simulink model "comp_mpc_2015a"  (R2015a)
settings: Solver=ode45  StartTime=0.0  StopTime=120  FixedStep=0.025  MaxStep=0.5  MinStep=0.03  RelTol=1e-6
InitFcn:
  | X_init
  | X_init2
  | Xinit_inter
StopFcn:
  | finalplot
  | finalplot2
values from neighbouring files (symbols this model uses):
  Xinit = [97004.3048907971    [X_init.m]
  Xinit2 = [155100    [X_init2.m]
libraries: simulink x4

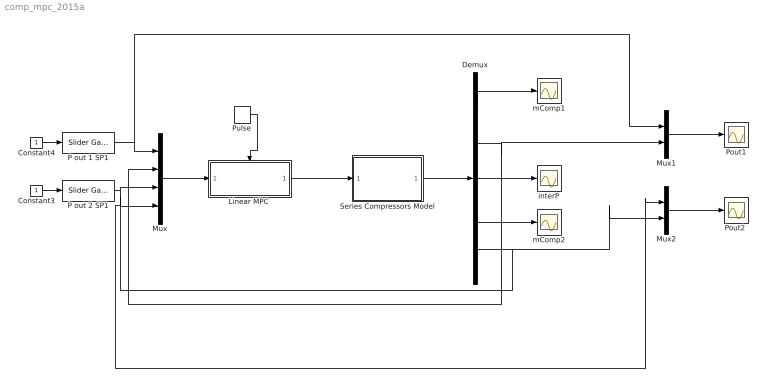
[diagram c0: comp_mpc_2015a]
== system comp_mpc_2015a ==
  Constant3 : Constant
  Constant4 : Constant
  Demux : Demux  Outputs=5
  "Linear MPC " : Subsystem  TreatAsAtomicUnit=on
  Mux : Mux
  Mux1 : Mux  Inputs=2
  Mux2 : Mux  Inputs=2
  P out 1 SP1 : simulink/Math Operations/Slider Gain  low=0  gain=173100  high=200000
  P out 2 SP1 : simulink/Math Operations/Slider Gain  low=0  gain=220000  high=2220000
  Pout1 : Scope
  "Pout2 " : Scope
  Pulse : DiscretePulseGenerator  PulseType=Time based  Period=0.5  PulseWidth=5
  Series Compressors Model : Subsystem
  interP : Scope
  mComp1 : Scope
  mComp2 : Scope
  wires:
  Demux/1 -> mComp1/1
  Demux/2 -> Mux1/2, Mux/2
  Demux/3 -> interP/1
  Demux/4 -> mComp2/1
  Demux/5 -> Mux2/2, Mux/4
  Pulse/1 -> "Linear MPC "/Trigger
  Mux/1 -> "Linear MPC "/1(In1)
  "Linear MPC "/1(Out1) -> Series Compressors Model/1(In1)
  Series Compressors Model/1(Out1) -> Demux/1
  Constant4/1 -> P out 1 SP1/1
  Constant3/1 -> P out 2 SP1/1
  P out 1 SP1/1 -> Mux1/1, Mux/1
  P out 2 SP1/1 -> Mux2/1, Mux/3
  Mux1/1 -> Pout1/1
  Mux2/1 -> "Pout2 "/1

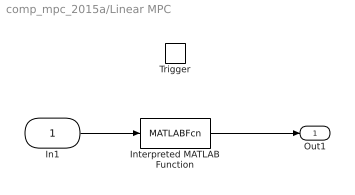
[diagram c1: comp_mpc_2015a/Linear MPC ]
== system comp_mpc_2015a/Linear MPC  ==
  In1 : Inport
  Trigger : TriggerPort
  Interpreted MATLAB Function : MATLABFcn  MATLABFcn=mpc_  Output1D=off
  Out1 : Outport
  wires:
  In1/1 -> Interpreted MATLAB Function/1
  Interpreted MATLAB Function/1 -> Out1/1

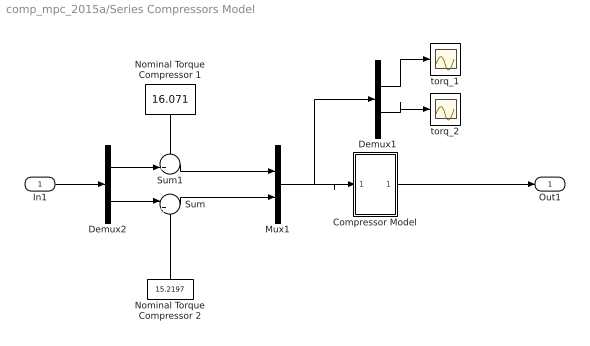
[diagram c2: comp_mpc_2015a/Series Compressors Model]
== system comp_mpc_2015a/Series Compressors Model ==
  In1 : Inport
  Compressor Model : Subsystem
  Demux1 : Demux  Outputs=2
  Demux2 : Demux  Outputs=2
  Mux1 : Mux  Inputs=2
  Nominal Torque Compressor 1 : Constant  Value=16.071
  Nominal Torque Compressor 2 : Constant  Value=15.2197
  Sum : Sum  Inputs=|++
  Sum1 : Sum  Inputs=++|
  torq_1 : Scope
  torq_2 : Scope
  Out1 : Outport
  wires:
  Demux1/2 -> torq_2/1
  Demux1/1 -> torq_1/1
  In1/1 -> Demux2/1
  Demux2/2 -> Sum/1
  Demux2/1 -> Sum1/2
  Sum/1 -> Mux1/2
  Sum1/1 -> Mux1/1
  Nominal Torque Compressor 1/1 -> Sum1/1
  Nominal Torque Compressor 2/1 -> Sum/2
  Mux1/1 -> Compressor Model/1(In1), Demux1/1
  Compressor Model/1(Out1) -> Out1/1

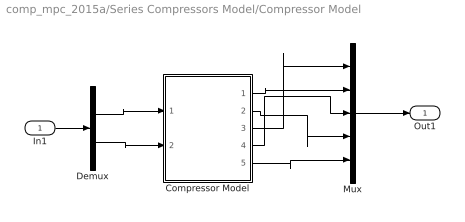
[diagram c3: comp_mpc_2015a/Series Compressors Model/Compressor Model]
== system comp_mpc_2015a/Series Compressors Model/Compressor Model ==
  In1 : Inport
  Compressor Model : Subsystem
  Demux : Demux  Outputs=2
  Mux : Mux  Inputs=5
  Out1 : Outport  PortDimensions=5
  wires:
  Compressor Model/4(iPres) -> Mux/3
  Mux/1 -> Out1/1
  Compressor Model/5(pout2) -> Mux/5
  Compressor Model/2(mcomp2) -> Mux/4
  Compressor Model/1(pout1) -> Mux/2
  Compressor Model/3(mcomp1) -> Mux/1
  Demux/1 -> Compressor Model/1(Torque 1)
  In1/1 -> Demux/1
  Demux/2 -> Compressor Model/2(torque 2)

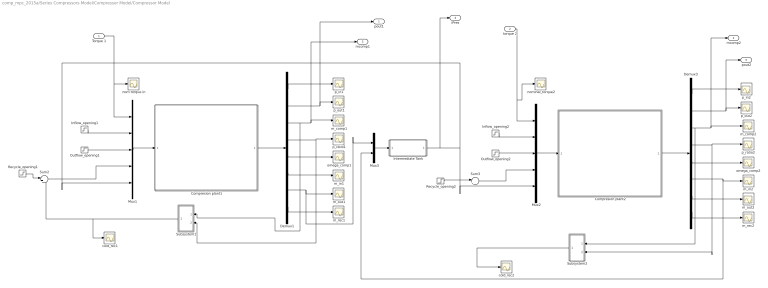
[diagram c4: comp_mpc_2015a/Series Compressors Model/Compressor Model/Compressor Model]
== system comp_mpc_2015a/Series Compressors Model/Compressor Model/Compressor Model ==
  Torque 1 : Inport
  torque 2 : Inport  Port=2
  Compresion plant1 : Subsystem
  Compresion plant2 : Subsystem
  Demux1 : Demux  Outputs=8
  Demux3 : Demux  Outputs=8
  Inflow_opening1 : Step  Time=0  Before=0.4541  After=0.4541  SampleTime=0
  Inflow_opening2 : Step  Time=25  Before=0.4541  After=0.4541  SampleTime=0
  Intermediate Tank : Subsystem
  Mux1 : Mux  Inputs=5
  Mux2 : Mux  Inputs=5
  Mux3 : Mux  Inputs=2
  Outflow_opening1 : Step  Time=10  Before=0.46  After=.29  SampleTime=0
  Outflow_opening2 : Step  Time=35  Before=0.46  After=.35  SampleTime=0
  Recycle_opening1 : Step  Time=2.05  After=0  SampleTime=0
  Recycle_opening2 : Step  Time=2.05  After=0  SampleTime=0
  Subsystem1 : Subsystem
  Subsystem2 : Subsystem
  Sum2 : Sum  Inputs=|++
  Sum3 : Sum  Inputs=|++
  cold_rec1 : Scope
  cold_rec2 : Scope
  m_comp1 : Scope
  m_comp2 : Scope
  m_in1 : Scope
  m_in2 : Scope
  m_out1 : Scope
  m_out2 : Scope
  m_rec1 : Scope
  m_rec2 : Scope
  nom torque in : Scope
  nominal_torque2 : Scope
  omega_comp1 : Scope
  omega_comp2 : Scope
  p_in1 : Scope
  p_in2 : Scope
  p_out1 : Scope
  p_out2 : Scope
  p_ratio1 : Scope
  p_ratio2 : Scope
  pout1 : Outport
  mcomp2 : Outport  Port=2
  mcomp1 : Outport  Port=3
  iPres : Outport  Port=4
  pout2 : Outport  Port=5
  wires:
  Sum3/1 -> Mux2/4
  Demux3/3 -> mcomp2/1, m_comp2/1, Subsystem2/1(In1)
  Demux3/4 -> Subsystem2/2(In2), p_ratio2/1
  Subsystem2/1(Out2) -> cold_rec2/1
  Torque 1/1 -> Mux1/1, nom torque in/1
  torque 2/1 -> Mux2/1, nominal_torque2/1
  Compresion plant1/1(Out1) -> Demux1/1
  Mux1/1 -> Compresion plant1/1(In1)
  Demux1/5 -> omega_comp1/1
  Demux1/6 -> m_in1/1
  Demux1/7 -> Mux3/1, m_out1/1
  Demux1/1 -> p_in1/1
  Demux1/2 -> pout1/1, p_out1/1
  Demux1/8 -> m_rec1/1
  Inflow_opening1/1 -> Mux1/2
  Compresion plant2/1(Out1) -> Demux3/1
  Mux2/1 -> Compresion plant2/1(In1)
  Demux3/5 -> omega_comp2/1
  Outflow_opening2/1 -> Mux2/3
  Demux3/6 -> Mux3/2, m_in2/1
  Demux3/7 -> m_out2/1
  Demux3/2 -> pout2/1, p_out2/1
  Demux3/8 -> m_rec2/1
  Outflow_opening1/1 -> Mux1/3
  Inflow_opening2/1 -> Mux2/2
  Mux3/1 -> Intermediate Tank/1(In1)
  Intermediate Tank/1(Out1) -> iPres/1, Mux2/5, Mux1/5
  Demux1/3 -> mcomp1/1, m_comp1/1, Subsystem1/1(In1)
  Demux1/4 -> p_ratio1/1, Subsystem1/2(In2)
  Subsystem1/1(Out2) -> Sum2/2, cold_rec1/1
  Recycle_opening1/1 -> Sum2/1
  Sum2/1 -> Mux1/4
  Recycle_opening2/1 -> Sum3/1
  Demux3/1 -> p_in2/1

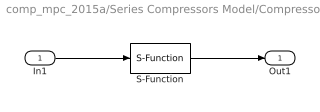
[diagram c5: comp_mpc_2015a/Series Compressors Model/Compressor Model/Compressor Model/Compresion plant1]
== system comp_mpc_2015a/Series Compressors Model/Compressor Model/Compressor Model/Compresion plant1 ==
  In1 : Inport
  S-Function : S-Function  FunctionName=comp_plant  Parameters=[],Xinit
  Out1 : Outport
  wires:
  S-Function/1 -> Out1/1
  In1/1 -> S-Function/1

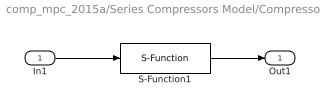
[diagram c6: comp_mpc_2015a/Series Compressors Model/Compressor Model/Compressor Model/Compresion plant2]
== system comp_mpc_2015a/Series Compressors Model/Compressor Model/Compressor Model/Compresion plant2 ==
  In1 : Inport
  S-Function1 : S-Function  FunctionName=comp_plant2  Parameters=[],Xinit2
  Out1 : Outport
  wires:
  S-Function1/1 -> Out1/1
  In1/1 -> S-Function1/1

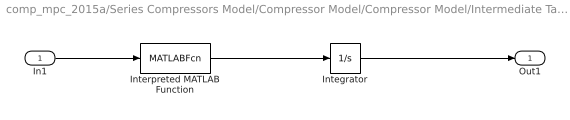
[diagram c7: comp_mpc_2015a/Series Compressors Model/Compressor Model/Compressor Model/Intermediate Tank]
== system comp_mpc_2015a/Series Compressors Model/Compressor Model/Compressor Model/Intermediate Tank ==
  In1 : Inport
  Integrator : Integrator  InitialCondition=155000
  Interpreted MATLAB Function : MATLABFcn  MATLABFcn=tank
  Out1 : Outport
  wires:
  In1/1 -> Interpreted MATLAB Function/1
  Interpreted MATLAB Function/1 -> Integrator/1
  Integrator/1 -> Out1/1

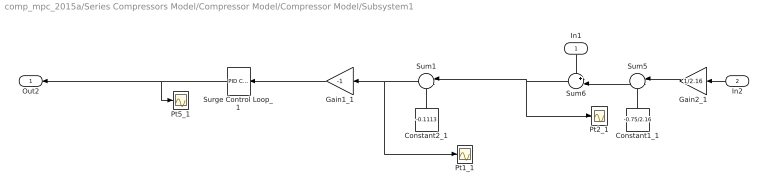
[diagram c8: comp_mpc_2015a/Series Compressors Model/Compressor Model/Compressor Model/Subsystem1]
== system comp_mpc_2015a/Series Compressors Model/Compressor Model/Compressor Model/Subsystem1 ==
  In1 : Inport
  In2 : Inport  Port=2
  Constant1_1 : Constant  Value=-0.75/2.16
  Constant2_1 : Constant  Value=-0.1113
  Gain1_1 : Gain  Gain=-1
  Gain2_1 : Gain  Gain=1/2.16
  Pt1_1 : Scope
  Pt2_1 : Scope
  Pt5_1 : Scope
  Sum1 : Sum  Inputs=|++
  Sum5 : Sum  Inputs=|++
  Sum6 : Sum  Inputs=+-|
  Surge Control Loop_1 : simulink/Continuous/PID Controller  Controller=PID  TimeDomain=Discrete-time  SampleTime=0.04  IntegratorMethod=Forward Euler  FilterMethod=Forward Euler  Form=Parallel  UseFilter=on  ControllerParametersSource=internal  P=0.8  I=2  D=0  N=2.82959055969234  InitialConditionSource=internal  InitialConditionForIntegrator=0  InitialConditionForFilter=0  ExternalReset=none  ZeroCross=off  LimitOutput=on  UpperSaturationLimit=1  LowerSaturationLimit=0  LinearizeAsGain=off  AntiWindupMode=back-calculation  Kb=1  TrackingMode=off  Kt=1  PParamMin=[]  PParamMax=[]  IParamMin=[]  IParamMax=[]  DParamMin=[]  DParamMax=[]  NParamMin=[]  NParamMax=[]  KbParamMin=[]  KbParamMax=[]  KtParamMin=[]  KtParamMax=[]  POutMin=[]  POutMax=[]  IOutMin=[]  IOutMax=[]  DOutMin=[]  DOutMax=[]  NOutMin=[]  NOutMax=[]  KbOutMin=[]  KbOutMax=[]  KtOutMin=[]  KtOutMax=[]  IntegratorOutMin=[]  IntegratorOutMax=[]  FilterOutMin=[]  FilterOutMax=[]  SumOutMin=[]  SumOutMax=[]  SumI1OutMin=[]  SumI1OutMax=[]  SumI2OutMin=[]  SumI2OutMax=[]  SumI3OutMin=[]  SumI3OutMax=[]  SumDOutMin=[]  SumDOutMax=[]  SaturationOutMin=[]  SaturationOutMax=[]  IntegratorContinuousStateAttributes=''  IntegratorStateMustResolveToSignalObject=off  IntegratorRTWStateStorageClass=Auto  FilterContinuousStateAttributes=''  FilterStateMustResolveToSignalObject=off  FilterRTWStateStorageClass=Auto  DifferentiatorICPrevScaledInput=0  DifferentiatorOutMin=[]  DifferentiatorOutMax=[]
  Out2 : Outport
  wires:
  Gain2_1/1 -> Sum5/1
  Constant1_1/1 -> Sum5/2
  Sum5/1 -> Sum6/2
  Sum6/1 -> Pt2_1/1, Sum1/1
  In2/1 -> Gain2_1/1
  Constant2_1/1 -> Sum1/2
  In1/1 -> Sum6/1
  Sum1/1 -> Pt1_1/1, Gain1_1/1
  Gain1_1/1 -> Surge Control Loop_1/1
  Surge Control Loop_1/1 -> Out2/1, Pt5_1/1

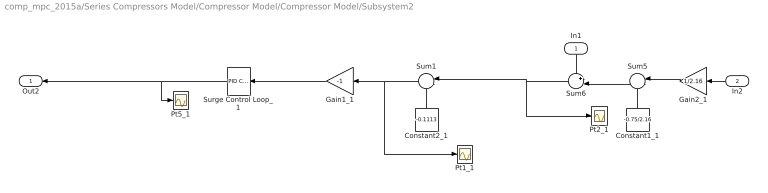
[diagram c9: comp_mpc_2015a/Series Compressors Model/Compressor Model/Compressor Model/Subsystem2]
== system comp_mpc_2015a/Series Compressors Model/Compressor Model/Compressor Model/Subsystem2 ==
  In1 : Inport
  In2 : Inport  Port=2
  Constant1_1 : Constant  Value=-0.75/2.16
  Constant2_1 : Constant  Value=-0.1113
  Gain1_1 : Gain  Gain=-1
  Gain2_1 : Gain  Gain=1/2.16
  Pt1_1 : Scope
  Pt2_1 : Scope
  Pt5_1 : Scope
  Sum1 : Sum  Inputs=|++
  Sum5 : Sum  Inputs=|++
  Sum6 : Sum  Inputs=+-|
  Surge Control Loop_1 : simulink/Continuous/PID Controller  Controller=PID  TimeDomain=Discrete-time  SampleTime=0.04  IntegratorMethod=Forward Euler  FilterMethod=Forward Euler  Form=Parallel  UseFilter=on  ControllerParametersSource=internal  P=0.8  I=2  D=0  N=2.82959055969234  InitialConditionSource=internal  InitialConditionForIntegrator=0  InitialConditionForFilter=0  ExternalReset=none  ZeroCross=off  LimitOutput=on  UpperSaturationLimit=1  LowerSaturationLimit=0  LinearizeAsGain=off  AntiWindupMode=back-calculation  Kb=1  TrackingMode=off  Kt=1  PParamMin=[]  PParamMax=[]  IParamMin=[]  IParamMax=[]  DParamMin=[]  DParamMax=[]  NParamMin=[]  NParamMax=[]  KbParamMin=[]  KbParamMax=[]  KtParamMin=[]  KtParamMax=[]  POutMin=[]  POutMax=[]  IOutMin=[]  IOutMax=[]  DOutMin=[]  DOutMax=[]  NOutMin=[]  NOutMax=[]  KbOutMin=[]  KbOutMax=[]  KtOutMin=[]  KtOutMax=[]  IntegratorOutMin=[]  IntegratorOutMax=[]  FilterOutMin=[]  FilterOutMax=[]  SumOutMin=[]  SumOutMax=[]  SumI1OutMin=[]  SumI1OutMax=[]  SumI2OutMin=[]  SumI2OutMax=[]  SumI3OutMin=[]  SumI3OutMax=[]  SumDOutMin=[]  SumDOutMax=[]  SaturationOutMin=[]  SaturationOutMax=[]  IntegratorContinuousStateAttributes=''  IntegratorStateMustResolveToSignalObject=off  IntegratorRTWStateStorageClass=Auto  FilterContinuousStateAttributes=''  FilterStateMustResolveToSignalObject=off  FilterRTWStateStorageClass=Auto  DifferentiatorICPrevScaledInput=0  DifferentiatorOutMin=[]  DifferentiatorOutMax=[]
  Out2 : Outport
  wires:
  Gain2_1/1 -> Sum5/1
  Constant1_1/1 -> Sum5/2
  Sum5/1 -> Sum6/2
  Sum6/1 -> Pt2_1/1, Sum1/1
  In2/1 -> Gain2_1/1
  Constant2_1/1 -> Sum1/2
  In1/1 -> Sum6/1
  Sum1/1 -> Pt1_1/1, Gain1_1/1
  Gain1_1/1 -> Surge Control Loop_1/1
  Surge Control Loop_1/1 -> Out2/1, Pt5_1/1
